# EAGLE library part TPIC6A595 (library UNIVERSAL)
8x otvoreny kolektor ovladany SPI zbernicou.
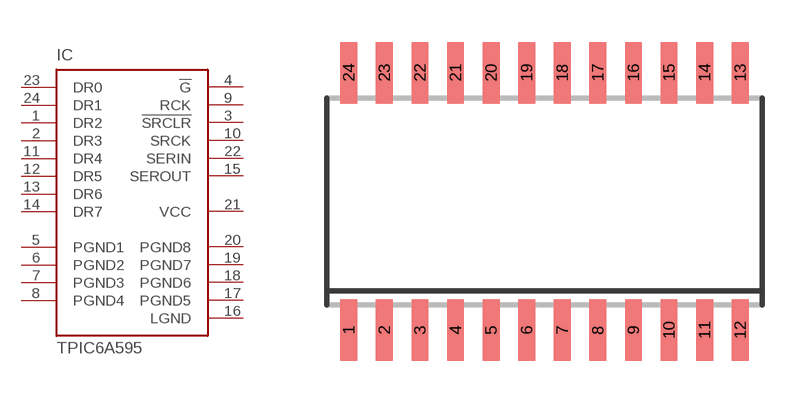
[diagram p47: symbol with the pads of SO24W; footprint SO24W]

Designator prefix IC

## TPIC6A595 (IC: TPIC6A595DW)  [SO24W]
1  DR2
2  DR3
3  !SRCLR  in
4  !G  in
5  PGND1  pwr
6  PGND2  pwr
7  PGND3  pwr
8  PGND4  pwr
9  RCK  in
10  SRCK  in
11  DR4
12  DR5
13  DR6
14  DR7
15  SEROUT  out
16  LGND  pwr
17  PGND5  pwr
18  PGND6  pwr
19  PGND7  pwr
20  PGND8  pwr
21  VCC  pwr
22  SERIN  in
23  DR0
24  DR1

## Footprint SO24W (pad centres in mm)
smd 0.6 x 2.2: 1 0.635,-0.79; 2 1.905,-0.79; 3 3.175,-0.79; 4 4.445,-0.79; 5 5.715,-0.79; 6 6.985,-0.79; 7 8.255,-0.79; 8 9.525,-0.79; 9 10.795,-0.79; 10 12.065,-0.79; 11 13.335,-0.79; 12 14.605,-0.79; 13 14.605,8.41; 14 13.335,8.41; 15 12.065,8.41; 16 10.795,8.41; 17 9.525,8.41; 18 8.255,8.41; 19 6.985,8.41; 20 5.715,8.41; 21 4.445,8.41; 22 3.175,8.41; 23 1.905,8.41; 24 0.635,8.41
